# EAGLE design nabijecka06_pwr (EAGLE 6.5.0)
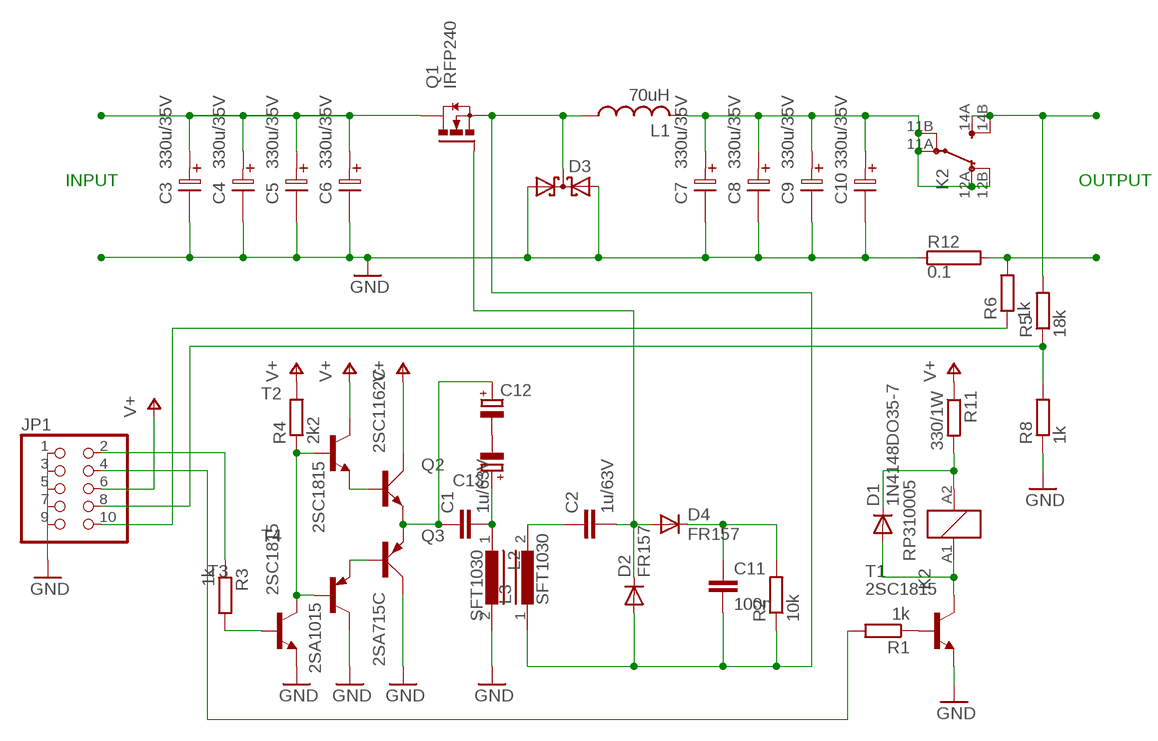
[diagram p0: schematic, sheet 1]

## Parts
C1  1u/63V  C-EU025-050X050  [C025-050X050]
C2  1u/63V  C-EU025-050X050  [C025-050X050]
C3  330u/35V  ELYT100  [ELYT100]
C4  330u/35V  ELYT100  [ELYT100]
C5  330u/35V  ELYT100  [ELYT100]
C6  330u/35V  ELYT100  [ELYT100]
C7  330u/35V  ELYT100  [ELYT100]
C8  330u/35V  ELYT100  [ELYT100]
C9  330u/35V  ELYT100  [ELYT100]
C10  330u/35V  ELYT100  [ELYT100]
C11  100n  C-EU050-024X044  [C050-024X044]
C12  CPOL-EUE2.5-7  [E2,5-7]
C13  CPOL-EUE2.5-7  [E2,5-7]
D1  1N4148DO35-7  [DO35-7]
D2  FR157  1N4004  [DO41-10]
D3  DIODE_2SCHOTTKY-SOT93V  [SOT93S]
D4  FR157  1N4004  [DO41-10]
JP1  PINHD-2X5  [2X05]
K2  RP310005  [RT-C/O16A5]
L1  70uH  L-USTJ7-U1  [TJ7-U1]
L2  SFT1030  [SFT1030]
L3  SFT1030  [SFT1030]
Q1  IRFP240  [TO247BV]
Q2  2SC1162C  BD139  [TO126AV]
Q3  2SA715C  BD140  [TO126AV]
R1  1k  R-EU_0204/7  [0204/7]
R2  10k  R-EU_0204/7  [0204/7]
R3  1k  R-EU_0204/7  [0204/7]
R4  2k2  R-EU_0204/7  [0204/7]
R5  18k  R-EU_0204/7  [0204/7]
R6  1k  R-EU_0204/7  [0204/7]
R8  1k  R-EU_0204/7  [0204/7]
R11  330/1W  R-EU_0309/12  [0309/12]
R12  0.1  RKH214-8  [KH214-8]
T1  2SC1815  [TO92-ECB]
T2  2SC1815  [TO92-ECB]
T3  2SC1815  [TO92-ECB]
T4  2SA1015  -PNP-TO92-BCE  [TO92-BCE]

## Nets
GND: C3.2 C4.2 C5.2 C6.2 C7.2 C8.2 C9.2 C10.2 D3.A1 D3.A2 JP1.1 JP1.3 JP1.5 JP1.7 JP1.9 L2.2 Q3.C R8.1 R12.1 T1.E T3.E T4.C
N$1: R4.1 T2.B T3.C T4.B
N$3: D1.A K2.A1 T1.C
N$4: R1.1 T1.B
N$5: D1.C K2.A2 R11.2
N$6: R3.2 T3.B
N$7: C1.2 C13.+ L2.1
N$8: Q2.B T2.E
N$9: JP1.4 R1.2
N$10: JP1.8 R5.1 R8.2
N$11: JP1.10 R6.1
N$12: C1.1 C12.+ Q2.E Q3.E
N$13: C2.1 L3.2
N$14: C11.2 D2.A D3.C L1.1 L3.1 Q1.S R2.1
N$15: C2.2 D2.C D4.A Q1.G
N$16: C11.1 D4.C R2.2
N$18: JP1.2 R3.1
N$19: Q3.B T4.E
N$22: C12.- C13.-
N$24: C7.1 C8.1 C9.1 C10.1 K2.11A(2:PA) K2.11B(2:PB) K2.12A(2:OA) K2.12B(2:OB) L1.2
OUT+: K2.14A(2:SA) K2.14B(2:SB) R5.2
OUT-: R6.2 R12.2
V+: JP1.6 Q2.C R4.2 R11.1 T2.C
VIN: C3.1 C4.1 C5.1 C6.1 Q1.D

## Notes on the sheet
- INPUT | OUTPUT

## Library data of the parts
C1 C2 C11 = rcl:C-EU: CAPACITOR, European symbol
C3-C10 = LAMPY02:ELYT100
C12 C13 = rcl:CPOL-EU: POLARIZED CAPACITOR, European symbol
D1 = diode:1N4148: DIODE
D2 D4 = diode:1N4004: DIODE
D3 = diode:DIODE_2SCHOTTKY-: Dual SCHOTTKY DIODE common cathode
JP1 = pinhead:PINHD-2X5: PIN HEADER
K2 = relay:RP?1*: Power PCB Relay RP II/1 SCHRACK 1 pole 16 A Source: http://www.schrack.com/.. 5834.pdf; MPN: RP310005; OC_FARNELL: unknown; OC_NEWARK: 48M7769
L1 = rcl:L-US: INDUCTOR, American symbol
L2 L3 = inductors:SFT1030: INDUCTOR
Q1 = transistor-power:IRFP240: HEXFET Power MosFet Source: http://www.irf.com/
Q2 = transistor-power:BD139: NPN TRANSISTOR
Q3 = transistor-power:BD140: PNP TRANSISTOR
R1-R6 R8 R11 = rcl:R-EU_: RESISTOR, European symbol
R12 = resistor-power:R: Power Resitor; OC_FARNELL: unknown; OC_NEWARK: unknown
T1-T3 = transistor:2SC1815: NPN EPITAXIAL TRANSISTOR Source: TOSHIBA .. 2SC1815 1.pdf
T4 = transistor-neu-to92:*-PNP-: PNP Transistror

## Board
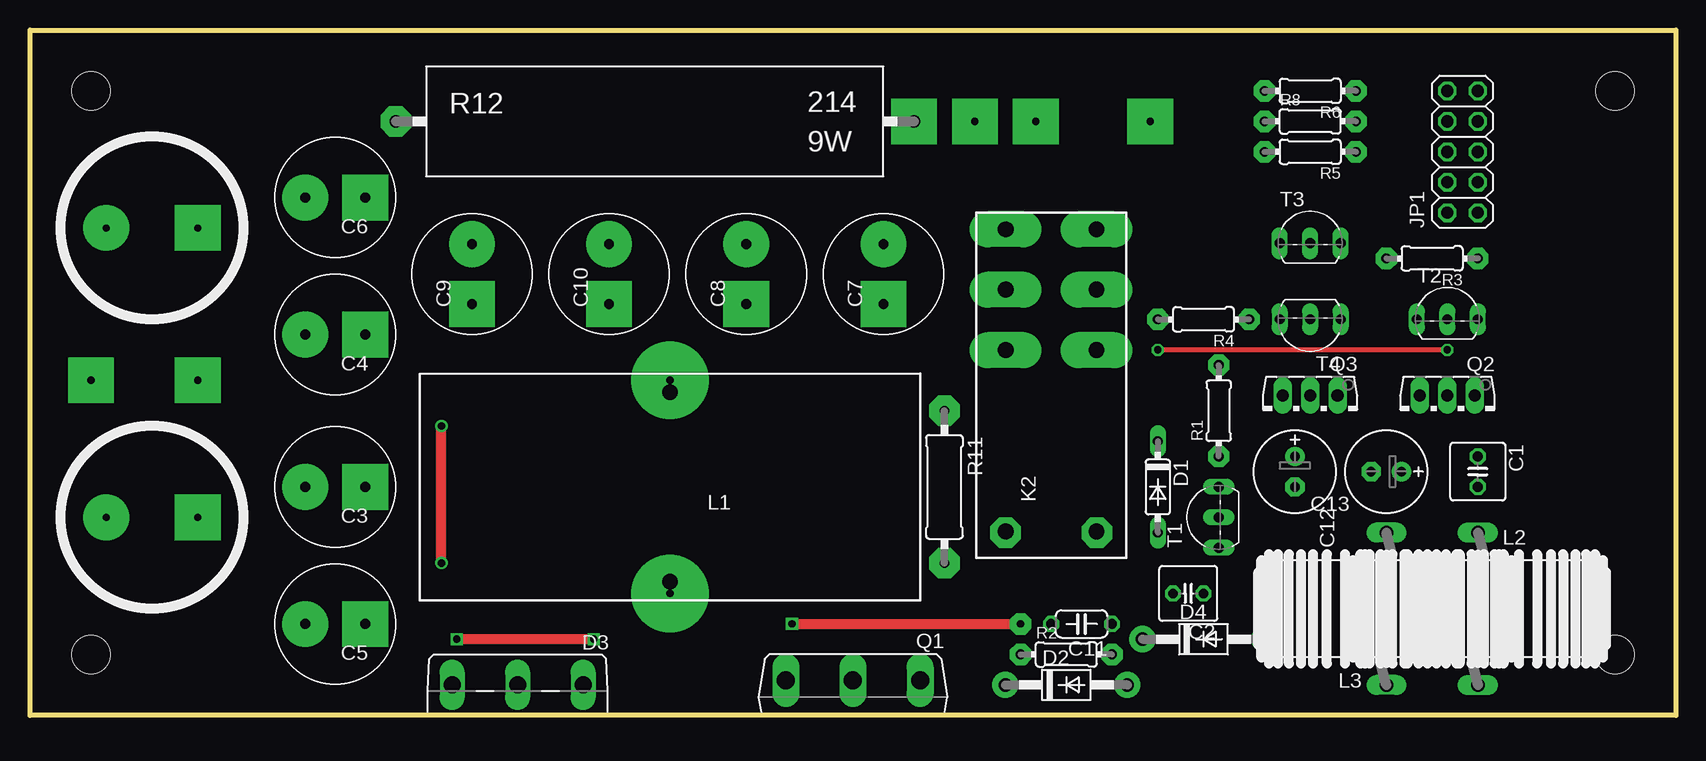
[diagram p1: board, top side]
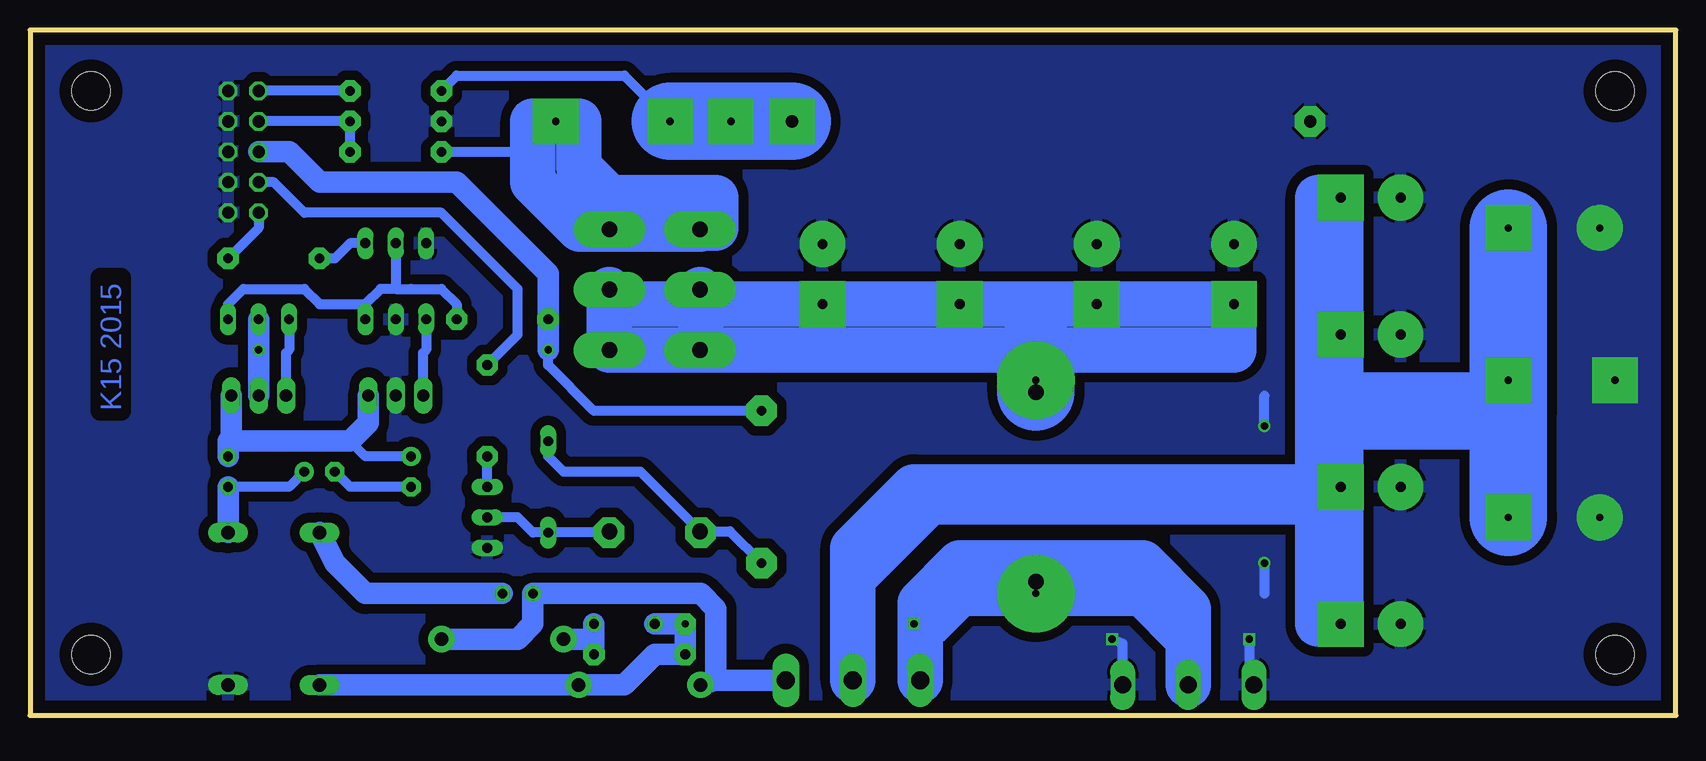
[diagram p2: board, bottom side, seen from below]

Size 137.16 x 57.15 mm. Coordinates in mm from the lower left corner, seen from the top.
Outline: 0,0 0,57.15 137.16,57.15 137.16,0 0,0
Copper layers (1*16): Top 0.035mm / dielectric 1.5mm / Bottom 0.035mm
Design rules "default": minimum track width 10mil, minimum drill 24mil, track to track 8mil, track to pad 8mil, pad to pad 8mil, via to via 8mil, smd to smd 8mil, copper to edge 40mil, drill to drill 8mil, minimum pad ring 10mil, minimum via ring 8mil, stop-mask expansion 4mil, vias tented up to drill 0mil, thermal gap 10mil
Holes 3.2 mm at 5.08,52.07 5.08,5.08 132.08,5.08 132.08,52.07

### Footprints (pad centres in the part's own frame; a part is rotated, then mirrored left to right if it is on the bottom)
C025-050X050 = drill 0.813 octagon: 1 -1.27,0; 2 1.27,0
ELYT100 = drill 0.813 pad 3.81 square: 1 -2.54,0 | drill 0.813 pad 3.81: 2 2.46,0
C050-024X044 = drill 0.813 octagon: 1 -2.54,0; 2 2.54,0
E2,5-7 = drill 0.813 pad 1.6: + -1.27,0 | drill 0.813 pad 1.6 octagon: - 1.27,0
DO35-7 = drill 0.813 long: A 3.81,0; C -3.81,0
DO41-10 = drill 1.118 pad 2.184: A 5.08,0; C -5.08,0
SOT93S = drill 1.397 long: A1 -5.461,-2.54; A2 5.461,-2.54; C 0,-2.54
2X05 = drill 1.016 octagon: 1 -5.08,-1.27; 2 -5.08,1.27; 3 -2.54,-1.27; 4 -2.54,1.27; 5 0,-1.27; 6 0,1.27; 7 2.54,-1.27; 8 2.54,1.27; 9 5.08,-1.27; 10 5.08,1.27
RT-C/O16A5 = drill 1.3 pad 3 long: 11A 7.56,3.78; 11B 7.56,-3.78; 12A 2.52,3.78; 12B 2.52,-3.78; 14A 12.6,3.78; 14B 12.6,-3.78 | drill 1.3: A1 -12.6,-3.78; A2 -12.6,3.78
TJ7-U1 = drill 1.3: 1 -7.9,0; 2 7.9,0
SFT1030 = drill 1.118 long: 1 -6.35,0; 2 6.35,0
TO247BV = drill 1.499 long: D 0,-2.921; G -5.588,-2.921; S 5.588,-2.921
TO126AV = drill 1.016 long: B 2.286,-1.27; C 0,-1.27; E -2.286,-1.27
0204/7 = drill 0.813 pad 1.778 octagon: 1 -3.81,0; 2 3.81,0
0309/12 = drill 0.813 pad 2.54 octagon: 1 -6.35,0; 2 6.35,0
KH214-8 = drill 1.016 pad 2.54 octagon: 1 -21.59,0; 2 21.59,0
TO92-ECB = drill 0.813 long: B 2.54,0; C 0,0; E -2.54,0
TO92-BCE = drill 0.813 long: B -2.54,0; C 0,0; E 2.54,0

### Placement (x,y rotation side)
C1  120.65,20.32 270 top
C2  96.52,10.16 180 top
C3  25.4,19.05 180 top
C4  25.4,31.75 180 top
C5  25.4,7.62 180 top
C6  25.4,43.18 180 top
C7  71.12,36.83 90 top
C8  59.69,36.83 90 top
C9  36.83,36.83 90 top
C10  48.26,36.83 90 top
C11  87.63,7.62 180 top
C12  105.41,20.32 270 top
C13  113.03,20.32 180 top
D1  93.98,19.05 270 top
D2  86.36,2.54 0 top
D3  40.64,0 180 top
D4  97.79,6.35 0 top
JP1  119.38,46.99 90 top
K2  85.09,27.94 90 top
L1  53.34,19.05 90 top
L2  120.65,8.89 270 top
L3  113.03,8.89 90 top
Q1  68.58,0 180 top
Q2  118.11,25.4 180 top
Q3  106.68,25.4 180 top
R1  99.06,25.4 90 top
R2  86.36,5.08 0 top
R3  116.84,38.1 180 top
R4  97.79,33.02 180 top
R5  106.68,46.99 180 top
R6  106.68,52.07 180 top
R8  106.68,49.53 0 top
R11  76.2,19.05 270 top
R12  52.07,49.53 0 top
T1  99.06,16.51 90 top
T2  118.11,33.02 0 top
T3  106.68,39.37 0 top
T4  106.68,33.02 180 top

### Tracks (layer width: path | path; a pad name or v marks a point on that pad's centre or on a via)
GND  (via drill 0.6, 0.6 pad 0.81, 0.6 pad 3.81)
  Top 0.813: v46.99,6.35 v35.56,6.35 | v34.29,12.7 v34.29,24.13
  Bottom 0.813: D3.A1 46.1,5.97 v46.99,6.35 | v35.56,6.35 35.56,2.92 D3.A2 | v34.29,12.7 34.29,10.16 | v34.29,24.13 34.29,26.67
  other vias: 5.08,27.94 6.35,40.64 6.35,16.51
  pour Bottom (isolate 0.813): 0,57.15 137.16,57.15 138.43,0 1.27,0
N$1
  Bottom 0.813: T3.C 106.68,35.56 | 106.68,35.56 107.95,35.56 109.22,34.29 | 109.22,34.29 T4.B | 106.68,35.56 105.41,35.56 102.87,35.56 101.6,34.29 R4.1 | T2.B 120.65,34.29 119.38,35.56 114.3,35.56 113.03,34.29 109.22,34.29
N$2
  Bottom 3.81: 91.44,49.53 91.44,45.72 88.9,43.18 80.01,43.18 80.01,40.64 82.55,40.64
N$3
  Bottom 0.813: K2.A1 88.97,15.24 D1.A 95.25,15.24 96.52,16.51 T1.C
N$4
  Bottom 0.813: T1.B R1.1
N$5
  Bottom 0.813: K2.A2 81.38,15.34 | D1.C 93.98,21.59 92.71,20.32 86.29,20.32 K2.A2 | R11.2 78.84,15.34 K2.A2
N$6
  Bottom 0.813: T3.B 110.49,39.37 111.76,38.1 R3.2
N$7
  Bottom 0.813: C13.+ 115.57,19.05 C1.2
  Bottom 1.778: L2.1 C1.2
N$8
  Bottom 0.813: T2.E 115.57,30.48 115.82,30.23 Q2.B
N$9
  Bottom 0.813: R1.2 96.52,31.75 96.52,35.56 102.87,41.91 114.3,41.91 116.84,44.45 JP1.4
N$10
  Bottom 0.813: R5.1 R8.2 JP1.8
N$11
  Bottom 0.813: R6.1 JP1.10
N$12
  Bottom 0.813: C12.+ 109.22,21.59 110.49,22.86
  Bottom 1.778: C1.1 120.65,22.86 | 120.65,22.86 110.49,22.86 108.97,24.38 Q3.E | Q2.E 120.4,23.11 120.65,22.86
N$13
  Bottom 1.778: C2.1 109.22,10.16 111.76,12.7 L3.2
N$14  (via drill 0.6, 0.6 pad 1.78, 0.6 pad 6.45)
  Top 0.813: v63.5,7.62 v82.55,7.62
  Bottom 0.813: Q1.S 62.99,7.11 v63.5,7.62
  Bottom 1.778: L3.1 D2.A 87.63,2.54 85.09,5.08 R2.1 v82.55,7.62 C11.2
  Bottom 3.81: D3.C 40.64,6.35 | 40.64,6.35 44.45,10.16 v53.34,10.16 | v53.34,10.16 59.69,10.16 62.23,7.62 | v53.34,10.16 L1.1 | 40.64,6.35 40.64,8.89 44.45,12.7 59.69,12.7 62.99,9.4 Q1.S
N$15
  Bottom 1.778: D4.A 96.52,6.35 95.25,7.62 C2.2 81.28,10.16 80.01,8.89 80.01,2.92 | Q1.G 80.01,2.92 | 80.01,2.92 D2.C
N$16
  Bottom 1.778: C11.1 R2.2 90.17,6.35 D4.C
N$17  (via drill 0.6 pad 2.54)
  other vias: 81.28,15.24
N$18
  Bottom 0.813: JP1.2 118.11,40.64 R3.1
N$19
  Bottom 0.813: T4.E 104.14,30.48 104.39,30.23 Q3.B
N$22
  Bottom 0.813: C12.- 110.49,19.05 C13.-
N$24  (via drill 0.6 pad 6.45)
  Bottom 3.81: 81.28,34.29 C7.1 C8.1 C10.1 C9.1 36.83,30.48 53.34,30.48 88.9,30.48 88.87,33.05 | 81.28,34.29 88.87,34.29 | 88.87,34.29 K2.11B | K2.11A 81.28,34.23 | K2.12A 81.28,31.73 81.28,34.23 | 81.28,34.23 81.28,34.29 | K2.12B 88.87,33.05 | 88.87,34.29 88.87,33.05
  Bottom 6.452: L1.2 v53.34,27.94 53.34,30.48
N$27  (via drill 0.6 pad 2.54)
  other vias: 88.9,15.24
OUT+  (via drill 0.6 pad 3.81)
  Bottom 0.813: R5.2 95.25,46.99 95.25,49.53
  Bottom 3.81: K2.14A K2.14B 91.34,40.54 95.25,44.45 95.25,49.53 v93.34,49.53
OUT-  (via drill 0.6 pad 3.81)
  Bottom 0.813: R6.2 101.6,53.34 87.63,53.34 v83.82,49.53
  Bottom 6.452: R12.2 v78.74,49.53 v83.82,49.53
  other vias: 73.66,49.53
V+  (via drill 0.6)
  Top 0.406: v118.11,30.48 v93.98,30.48
  Bottom 0.813: R11.1 90.17,25.4 93.98,29.21 v93.98,30.48
  Bottom 1.778: Q2.C v118.11,30.48 T2.C | v93.98,30.48 R4.2 93.98,36.83 101.6,44.45 113.03,44.45 115.57,46.99 JP1.6
VIN  (via drill 0.6 pad 3.81)
  Bottom 3.81: C6.1 C4.1 27.94,25.4 C3.1 27.94,17.78 | 27.94,17.78 C5.1 | Q1.D 68.58,11.43 | 68.58,11.43 62.23,17.78 27.94,17.78 | 68.58,11.43 68.58,13.97 63.5,19.05 29.84,19.05 | 29.84,19.05 29.84,7.62 | 29.84,19.05 29.84,43.18
  Bottom 6.452: 13.97,25.4 v13.97,27.94 v13.97,40.64 | 13.97,25.4 27.94,25.4 | v13.97,16.51 13.97,25.4

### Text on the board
Bottom: K15 2015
